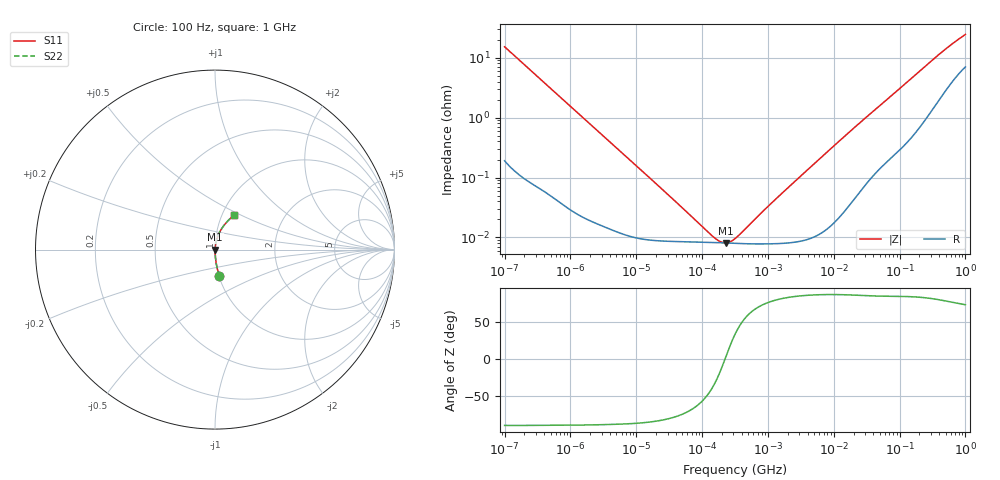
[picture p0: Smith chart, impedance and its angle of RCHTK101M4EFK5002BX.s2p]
! RCHTK101M4EFK5002BX  S-PARAMETER MODEL  (AEC-Q200 qualified)
! Model Generated by ELNA Corporation (http://www.ty-top.com)
! Version 1.0
! ELNA Control No. 240315
! Copyright (c) 2024 ELNA CO.,LTD. All Rights Reserved.
! Products Name : CONDUCTIVE POLYMER HYBRID ALUMINUM ELECTROLYTIC CAPACITORS
! Characteristics :
!  Capacitance  :  100uF  ,  Rated voltage  :  63V
!  Operating Temp. Range  :  -55 to +125 degC  ,  Endurance  :  6000hr at 125 degC
!  Dimension D  :  10mm  ,  Dimension L  :  12.5mm
! Frequency Range : 100Hz - 1GHz
! External Node Assignments :
!  1  o---| |---o  2
# MHz S RI R 50
!Freq[MHz].  S11 Real  S11 Imag  S21 Real  S21 Imag  S12 Real  S12 Imag  S22 Real  S22 Imag
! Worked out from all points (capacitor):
!   401 points, 100 Hz to 1 GHz, reference 50 ohm
!   read as one part in series: C = 105 uF near 108 Hz
!   lowest |Z| = 8.11 mohm at 229.1 kHz (marker M1)
!   series resonance near 222.7 kHz, so ESL is about 4.9 nH
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0.0001  0.0244 -0.1482  0.9756 0.1482  0.9756 0.1482  0.0244 -0.1482
0.000113  0.0194 -0.132  0.9806 0.132  0.9806 0.132  0.0194 -0.132
0.000183  0.00789 -0.0825  0.9921 0.0825  0.9921 0.0825  0.00789 -0.0825
0.000309  0.00314 -0.0493  0.9969 0.0493  0.9969 0.0493  0.00314 -0.0493
0.000613  0.00105 -0.0251  0.9989 0.0251  0.9989 0.0251  0.00105 -0.0251
0.001488  0.00033 -0.0104  0.9997 0.0104  0.9997 0.0104  0.00033 -0.0104
0.022131  8.84e-05 -0.000708  0.9999 0.000708  0.9999 0.000708  8.84e-05 -0.000708
0.141254  8.28e-05 -6.8e-05  0.9999 6.8e-05  0.9999 6.8e-05  8.28e-05 -6.8e-05
0.153109  8.26e-05 -5.54e-05  0.9999 5.54e-05  0.9999 5.54e-05  8.26e-05 -5.54e-05
0.165959  8.23e-05 -4.32e-05  0.9999 4.32e-05  0.9999 4.32e-05  8.23e-05 -4.32e-05
0.229087  8.1e-05 4.14e-06  0.9999 -4.14e-06  0.9999 -4.14e-06  8.1e-05 4.14e-06
0.316228  7.98e-05 5.27e-05  0.9999 -5.27e-05  0.9999 -5.27e-05  7.98e-05 5.27e-05
0.342768  7.95e-05 6.57e-05  0.9999 -6.57e-05  0.9999 -6.57e-05  7.95e-05 6.57e-05
0.371535  7.93e-05 7.91e-05  0.9999 -7.91e-05  0.9999 -7.91e-05  7.93e-05 7.91e-05
1.059254  7.84e-05 0.000341  0.9999 -0.000341  0.9999 -0.000341  7.84e-05 0.000341
4.704354  0.000101 0.00158  0.9999 -0.00158  0.9999 -0.00158  0.000101 0.00158
20.06781  0.000468 0.00663  0.9995 -0.00663  0.9995 -0.00663  0.000468 0.00663
69.9842  0.00245 0.0215  0.9975 -0.0215  0.9975 -0.0215  0.00245 0.0215
176.8072  0.00834 0.0516  0.9917 -0.0516  0.9917 -0.0516  0.00834 0.0516
395.8221  0.0307 0.1059  0.9693 -0.1059  0.9693 -0.1059  0.0307 0.1059
668.3439  0.0669 0.155  0.9331 -0.155  0.9331 -0.155  0.0669 0.155
1000  0.1081 0.1948  0.8919 -0.1948  0.8919 -0.1948  0.1081 0.1948
